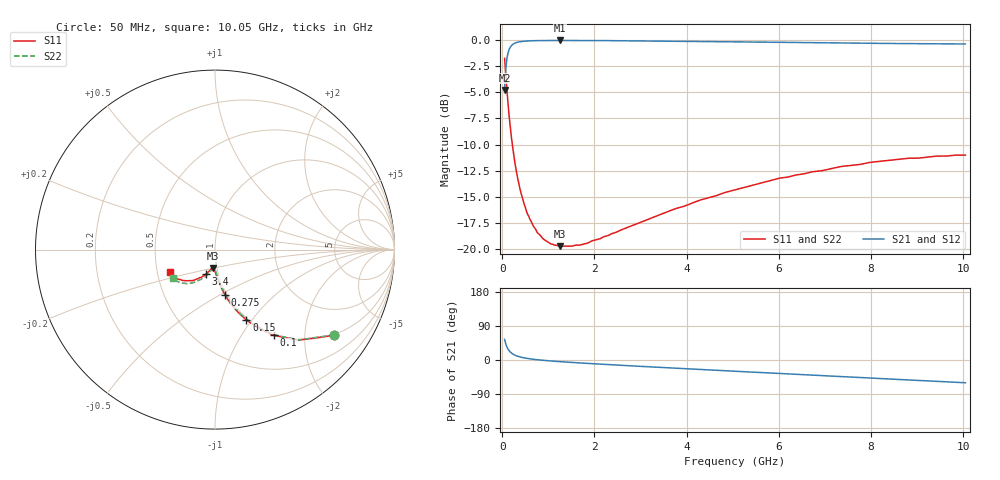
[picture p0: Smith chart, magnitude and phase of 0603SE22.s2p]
! AVX Thin Film Operation		Date: August 2001
! Description: Accu-P® Series, Thin Film, SMD, RF Capacitor
! Part Number: 06033J220FBT
! 50 MHz  -  10.05 GHz
! Serial Measurements
# mhz S db R 50
!	S11		S21		S12		S22
!	dB	Phase	dB	Phase	dB	Phase	dB	Phase
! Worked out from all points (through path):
!   401 points, 50 MHz to 10.05 GHz, reference 50 ohm
!   highest |S21| = -0.05 dB at 1.25 GHz (marker M1); lowest = -4.8 dB at 50 MHz (marker M2)
!   group delay of S21, straight-line fit = 18.9 ps
!   lowest |S11| = -19.7 dB at 1.25 GHz (marker M3), VSWR 1.23, Z = 48 - j10 ohm
!   |S11| at or under -10 dB: 218 MHz to end of sweep
!   |S22| runs from -19.7 to -1.8 dB; largest |S21 - S12| = 0
!   S11 on the Smith chart (normalised r, x): 50 MHz: 0.97, -2.79; 100 MHz: 0.98, -1.40; 150 MHz: 0.98, -0.94; 275 MHz: 0.98, -0.53; 3.4 GHz: 0.87, -0.24; 10.05 GHz: 0.58, -0.16
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50  -1.76 -35.8  -4.77 54.3  -4.77 54.3  -1.76 -35.6
100  -4.75 -55.6  -1.77 34.5  -1.77 34.5  -4.75 -55.3
125  -6.13 -61.5  -1.22 28.6  -1.22 28.6  -6.13 -61.2
150  -7.35 -66.0  -0.89 24.2  -0.89 24.2  -7.35 -65.5
175  -8.41 -69.3  -0.68 20.9  -0.68 20.9  -8.41 -68.8
200  -9.39 -72.0  -0.54 18.2  -0.54 18.2  -9.39 -71.4
275  -11.78 -77.5  -0.30 12.7  -0.30 12.7  -11.78 -76.8
350  -13.55 -81.1  -0.20 9.2  -0.20 9.2  -13.55 -80.1
425  -14.92 -83.6  -0.15 6.8  -0.15 6.8  -14.92 -82.4
525  -16.37 -86.0  -0.11 4.5  -0.11 4.5  -16.37 -84.6
650  -17.55 -88.4  -0.08 2.2  -0.08 2.2  -17.55 -86.7
800  -18.56 -90.5  -0.07 0.2  -0.07 0.2  -18.56 -88.6
925  -19.12 -92.0  -0.06 -1.2  -0.06 -1.2  -19.12 -90.0
1075  -19.50 -93.5  -0.05 -2.7  -0.05 -2.7  -19.50 -91.3
1250  -19.70 -95.2  -0.05 -4.3  -0.05 -4.3  -19.70 -92.8
1725  -19.55 -99.0  -0.06 -8.1  -0.06 -8.1  -19.45 -96.4
2275  -18.72 -103.0  -0.07 -12.0  -0.07 -12.0  -18.72 -99.9
3400  -16.73 -110.9  -0.10 -19.3  -0.10 -19.3  -16.73 -106.9
5050  -14.32 -121.4  -0.18 -29.7  -0.18 -29.7  -14.32 -117.4
6725  -12.60 -132.0  -0.26 -39.8  -0.26 -39.8  -12.60 -127.0
8400  -11.49 -143.1  -0.34 -50.1  -0.34 -50.1  -11.49 -136.2
10050  -11.00 -153.6  -0.39 -60.0  -0.39 -60.0  -10.92 -145.8
